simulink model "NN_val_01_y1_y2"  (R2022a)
settings: Solver=VariableStepAuto  StartTime=0.0  StopTime=300  RelTol=1e-3
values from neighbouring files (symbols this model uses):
  C = 6.3000e-04    (= 0.00063)    [maglev_init.m]
  g = 9.80    (= 9.8)    [maglev_init.m]
  K = 1.0e+03 * [-2.4567   -0.1235    0.0237]    [maglev_init.m]
  L1 = 0.6000    (= 0.6)    [maglev_init.m]
  m = 0.0300    (= 0.03)    [maglev_init.m]
  mpert = 0    [maglev_init.m]
  R = 45    [maglev_init.m]
  Ts = 0.005    [maglev_init.m]    (also in train_net.m)
  x1_0 = 0.1    [maglev_init.m]
  x1_d = 0.05    [maglev_init.m]
  x2_0 = 0    [maglev_init.m]
  x2_d = 0    [maglev_init.m]
  x3_0 = 0.2    [maglev_init.m]
undefined symbols (not defined in the file or in its folder): magnitude
libraries: neural x26

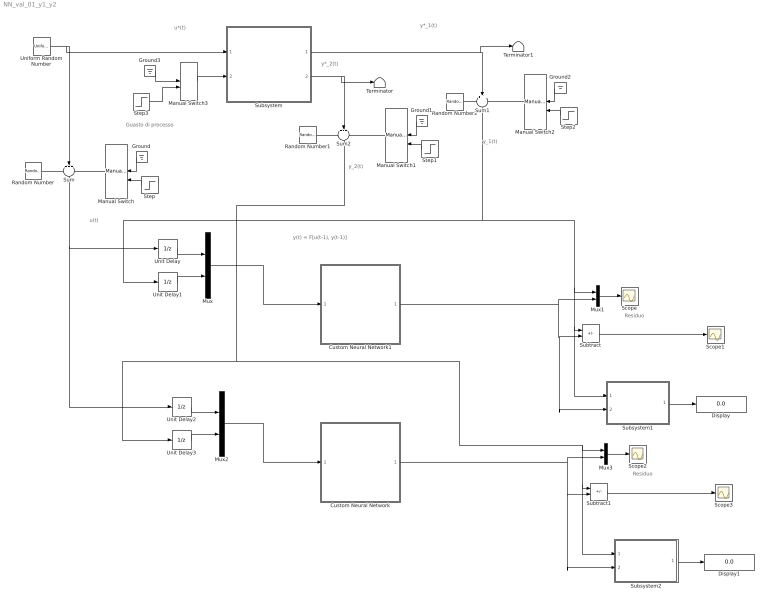
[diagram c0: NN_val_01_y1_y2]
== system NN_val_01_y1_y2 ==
  note: Residuo
  note: y(t) = F[u(t-1), y(t-1)]
  note: y_2(t)
  note: y*_1(t)
  note: u(t)
  note: y*_2(t)
  note: y_1(t)
  note: u*(t)
  note: Guasto di processo
  note: Residuo
  Custom Neural Network : Subsystem
      mask help: Custom Neural Network
  Custom Neural Network1 : Subsystem
      mask help: Custom Neural Network
  Display : Display
  Display1 : Display
  Ground{,1..3} (4 alike) : Ground
  Manual Switch : ManualSwitch
  Manual Switch1 : ManualSwitch  CurrentSetting=0
  Manual Switch2 : ManualSwitch
  Manual Switch3 : ManualSwitch
  Mux{,1..3} (4 alike) : Mux  Inputs=2
  Random Number : RandomNumber  Variance=1e-9  Seed=1  SampleTime=Ts
  Random Number1 : RandomNumber  Variance=1e-6  Seed=3  SampleTime=Ts
  Random Number2 : RandomNumber  Variance=1e-9  Seed=2  SampleTime=Ts
  Scope{,1..3} (4 alike) : Scope
  Step : Step  Time=150  SampleTime=0
  Step1 : Step  Time=150  SampleTime=0
  Step2 : Step  Time=150  SampleTime=0
  Step3 : Step  Time=15  After=2*R  SampleTime=0
  Subsystem : Subsystem
  Subsystem1 : Subsystem
  Subsystem2 : Subsystem
  Subtract : Sum  Inputs=+-
  Subtract1 : Sum  Inputs=+-
  Sum : Sum  Inputs=+++
  Sum1 : Sum  Inputs=+++
  Sum2 : Sum  Inputs=+++
  Terminator : Terminator
  Terminator1 : Terminator
  Uniform Random Number : UniformRandomNumber  Minimum=x1_d*0.9  Maximum=x1_d*1.1  Seed=1  SampleTime=0.5
  Unit Delay{,1..3} (4 alike) : UnitDelay  SampleTime=Ts  HasFrameUpgradeWarning=on
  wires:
  Subsystem/1(Out1) -> Terminator1/1, Sum1/2
  Subsystem/2(Out2) -> Terminator/1, Sum2/2
  Random Number/1 -> Sum/1
  Manual Switch/1 -> Sum/3
  Manual Switch2/1 -> Sum1/3
  Manual Switch1/1 -> Sum2/3
  Random Number1/1 -> Sum2/1
  Ground/1 -> Manual Switch/1
  Step/1 -> Manual Switch/2
  Ground1/1 -> Manual Switch1/1
  Step1/1 -> Manual Switch1/2
  Random Number2/1 -> Sum1/1
  Ground2/1 -> Manual Switch2/1
  Step2/1 -> Manual Switch2/2
  Manual Switch3/1 -> Subsystem/2(fs)
  Ground3/1 -> Manual Switch3/1
  Uniform Random Number/1 -> Subsystem/1(u), Sum/2
  Step3/1 -> Manual Switch3/2
  Sum/1 -> Unit Delay2/1, Unit Delay/1
  Unit Delay/1 -> Mux/1
  Unit Delay1/1 -> Mux/2
  Mux/1 -> Custom Neural Network1/1(Input)
  Custom Neural Network1/1(Output) -> Mux1/2, Subsystem1/2(y_prev), Subtract/2
  Subtract/1 -> Scope1/1
  Mux1/1 -> Scope/1
  Sum1/1 -> Subsystem1/1(y_mis), Subtract/1, Mux1/1, Unit Delay1/1
  Subsystem1/1(VAF%) -> Display/1
  Mux2/1 -> Custom Neural Network/1(Input)
  Unit Delay2/1 -> Mux2/1
  Unit Delay3/1 -> Mux2/2
  Subtract1/1 -> Scope3/1
  Custom Neural Network/1(Output) -> Mux3/2, Subsystem2/2(y_prev), Subtract1/2
  Mux3/1 -> Scope2/1
  Subsystem2/1(VAF%) -> Display1/1
  Sum2/1 -> Subsystem2/1(y_mis), Subtract1/1, Mux3/1, Unit Delay3/1

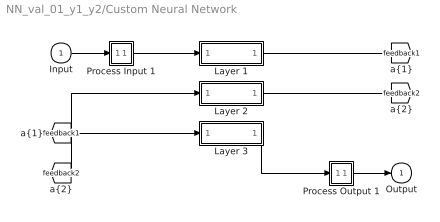
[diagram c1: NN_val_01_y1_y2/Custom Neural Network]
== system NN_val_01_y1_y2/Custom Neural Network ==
  Input : Inport  PortDimensions=2  SampleTime=0.005
  Layer 1 : Subsystem
  Layer 2 : Subsystem
  Layer 3 : Subsystem
  Process Input 1 : Subsystem
  Process Output 1 : Subsystem
  Output : Outport  InitialOutput=0
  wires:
  Input/1 -> Process Input 1/1(x)
  Process Output 1/1(y) -> Output/1
  Process Input 1/1(p) -> Layer 1/1("p{1}")
  Layer 1/1("a{1}") -> [feedback1]
  [feedback1] -> Layer 2/1("a{1} ")
  Layer 2/1("a{2}") -> [feedback2]
  [feedback2] -> Layer 3/1("a{2} ")
  Layer 3/1("a{3}") -> Process Output 1/1(a)

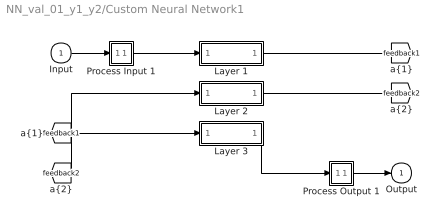
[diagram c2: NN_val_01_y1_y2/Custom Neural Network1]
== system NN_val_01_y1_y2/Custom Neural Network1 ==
  Input : Inport  PortDimensions=2  SampleTime=0.005
  Layer 1 : Subsystem
  Layer 2 : Subsystem
  Layer 3 : Subsystem
  Process Input 1 : Subsystem
  Process Output 1 : Subsystem
  Output : Outport  InitialOutput=0
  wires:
  Layer 3/1("a{3}") -> Process Output 1/1(a)
  [feedback2] -> Layer 3/1("a{2} ")
  Layer 2/1("a{2}") -> [feedback2]
  [feedback1] -> Layer 2/1("a{1} ")
  Layer 1/1("a{1}") -> [feedback1]
  Process Input 1/1(p) -> Layer 1/1("p{1}")
  Process Output 1/1(y) -> Output/1
  Input/1 -> Process Input 1/1(x)

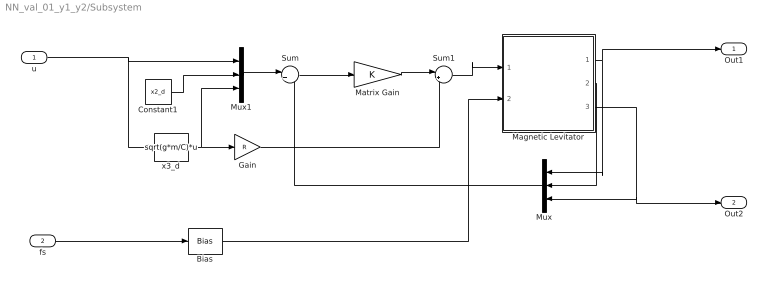
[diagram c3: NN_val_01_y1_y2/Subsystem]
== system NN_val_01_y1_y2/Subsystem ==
  u : Inport
  fs : Inport  Port=2
  Bias : Bias  Bias=R
  Constant1 : Constant  Value=x2_d
  Gain : Gain  Gain=R
  Magnetic Levitator : Subsystem  mask{m=m+mpert, R=R, L1=L1, C=C, g=g}
      mask prompts: m "ball's mass (m)"; R "Electromagnet's resistance (R)"; L1 "Electromagnet's inductance (L1)"; C "Magnetic force constant (C)"; g "Gravitational acceleration (g)"
  Matrix Gain : Gain  Gain=K  Multiplication=Matrix(K*u)  SaturateOnIntegerOverflow=on
  Mux : Mux  Inputs=3
  Mux1 : Mux  Inputs=3
  Sum : Sum  Inputs=|+-  InputSameDT=on  SaturateOnIntegerOverflow=on
  Sum1 : Sum  Inputs=|++  InputSameDT=on  SaturateOnIntegerOverflow=on
  x3_d : Fcn  Expr=sqrt(g*m/C)*u
  Out1 : Outport
  Out2 : Outport  Port=2
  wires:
  u/1 -> x3_d/1, Mux1/1
  Magnetic Levitator/2(x2) -> Mux/2
  x3_d/1 -> Mux1/3, Gain/1
  Mux1/1 -> Sum/1
  Gain/1 -> Sum1/2
  Mux/1 -> Sum/2
  Constant1/1 -> Mux1/2
  Sum/1 -> Matrix Gain/1
  Sum1/1 -> Magnetic Levitator/1(u)
  Magnetic Levitator/1(x1) -> Out1/1, Mux/1
  Magnetic Levitator/3(x3) -> Out2/1, Mux/3
  Matrix Gain/1 -> Sum1/1
  Bias/1 -> Magnetic Levitator/2(fs)
  fs/1 -> Bias/1

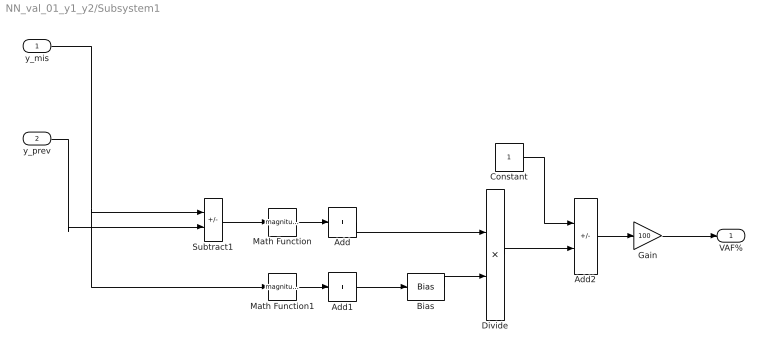
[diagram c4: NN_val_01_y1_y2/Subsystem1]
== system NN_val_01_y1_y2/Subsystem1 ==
  y_mis : Inport
  y_prev : Inport  Port=2
  Add : Sum  Inputs=+
  Add1 : Sum  Inputs=+
  Add2 : Sum  Inputs=+-
  Bias : Bias  Bias=1e-7
  Constant : Constant
  Divide : Product  Inputs=*/
  Gain : Gain  Gain=100
  Math Function : Math  Operator=magnitude^2
  Math Function1 : Math  Operator=magnitude^2
  Subtract1 : Sum  Inputs=+-
  VAF% : Outport
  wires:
  Add2/1 -> Gain/1
  Math Function/1 -> Add/1
  Bias/1 -> Divide/2
  y_mis/1 -> Math Function1/1, Subtract1/1
  Add1/1 -> Bias/1
  Math Function1/1 -> Add1/1
  Subtract1/1 -> Math Function/1
  Constant/1 -> Add2/1
  Divide/1 -> Add2/2
  Add/1 -> Divide/1
  y_prev/1 -> Subtract1/2
  Gain/1 -> VAF%/1

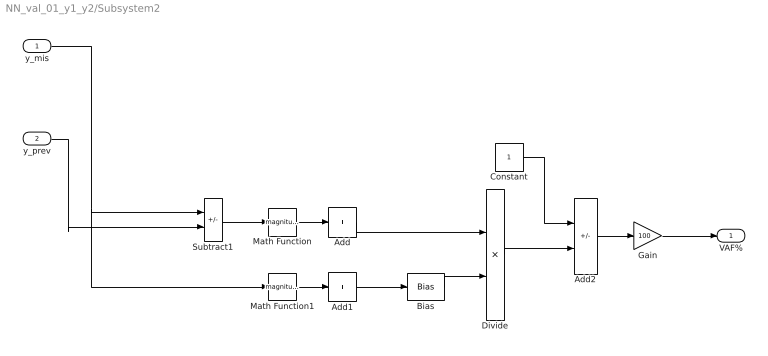
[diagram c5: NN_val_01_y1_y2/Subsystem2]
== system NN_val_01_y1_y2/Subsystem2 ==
  y_mis : Inport
  y_prev : Inport  Port=2
  Add : Sum  Inputs=+
  Add1 : Sum  Inputs=+
  Add2 : Sum  Inputs=+-
  Bias : Bias  Bias=1e-7
  Constant : Constant
  Divide : Product  Inputs=*/
  Gain : Gain  Gain=100
  Math Function : Math  Operator=magnitude^2
  Math Function1 : Math  Operator=magnitude^2
  Subtract1 : Sum  Inputs=+-
  VAF% : Outport
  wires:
  Add2/1 -> Gain/1
  Math Function/1 -> Add/1
  Bias/1 -> Divide/2
  y_mis/1 -> Math Function1/1, Subtract1/1
  Add1/1 -> Bias/1
  Math Function1/1 -> Add1/1
  Subtract1/1 -> Math Function/1
  Constant/1 -> Add2/1
  Divide/1 -> Add2/2
  Add/1 -> Divide/1
  y_prev/1 -> Subtract1/2
  Gain/1 -> VAF%/1

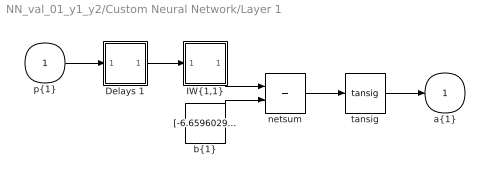
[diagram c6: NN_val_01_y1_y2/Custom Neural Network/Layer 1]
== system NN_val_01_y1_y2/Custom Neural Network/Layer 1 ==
  "p{1}" : Inport  PortDimensions=2  SampleTime=0.005
  Delays 1 : Subsystem
  "IW{1,1}" : Subsystem
  "b{1}" : Constant  Value=[-6.659602904330821360190384439192712306976318359375;3.45327763320656888623716440633870661258697509765625;1.7250442827917229493550621555186808109283447265625;0.2469389502636202549101795966635108925402164459228515625]
  netsum : Sum  Inputs=2  InputSameDT=on  SaturateOnIntegerOverflow=on
  tansig : neural/Transfer Functions/tansig
  "a{1}" : Outport  InitialOutput=[0;0;0;0]
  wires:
  "p{1}"/1 -> Delays 1/1("p{1}")
  Delays 1/1("pd{1,1}") -> "IW{1,1}"/1("pd{1,1}")
  "IW{1,1}"/1("iz{1,1}") -> netsum/1
  "b{1}"/1 -> netsum/2
  netsum/1 -> tansig/1
  tansig/1 -> "a{1}"/1

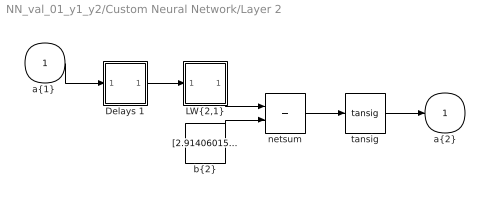
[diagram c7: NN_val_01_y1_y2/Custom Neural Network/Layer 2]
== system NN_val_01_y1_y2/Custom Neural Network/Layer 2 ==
  "a{1} " : Inport  PortDimensions=4  SampleTime=0.005
  Delays 1 : Subsystem
  "LW{2,1}" : Subsystem
  "b{2}" : Constant  Value=[2.914060157524335448187002839404158294200897216796875;-1.7057329147950757164409196775523014366626739501953125;-1.0860188396599046445345493339118547737598419189453125;-0.237937741106720890282844038665643893182277679443359375;-0.2127850090079609068904886726159020327031612396240234375;1.0101599307664710369891736263525672256946563720703125;1.8204085838934105368025484494864940643310546875;-2.778407191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
  netsum : Sum  Inputs=2  InputSameDT=on  SaturateOnIntegerOverflow=on
  tansig : neural/Transfer Functions/tansig
  "a{2}" : Outport  InitialOutput=[0;0;0;0;0;0;0;0]
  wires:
  "a{1} "/1 -> Delays 1/1("p{2}")
  Delays 1/1("pd{2,1}") -> "LW{2,1}"/1("ad{2,1}")
  "LW{2,1}"/1("lz{2,1}") -> netsum/1
  "b{2}"/1 -> netsum/2
  netsum/1 -> tansig/1
  tansig/1 -> "a{2}"/1

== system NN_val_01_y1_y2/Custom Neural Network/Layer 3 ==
  "a{2} " : Inport  PortDimensions=8  SampleTime=0.005
  Delays 1 : Subsystem
  "LW{3,2}" : Subsystem
  "b{3}" : Constant  Value=0.5176708554335636147669674755888991057872772216796875
  netsum : Sum  Inputs=2  InputSameDT=on  SaturateOnIntegerOverflow=on
  purelin : neural/Transfer Functions/purelin
  "a{3}" : Outport  InitialOutput=0
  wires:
  "a{2} "/1 -> Delays 1/1("p{3}")
  Delays 1/1("pd{3,2}") -> "LW{3,2}"/1("ad{3,2}")
  "LW{3,2}"/1("lz{3,2}") -> netsum/1
  "b{3}"/1 -> netsum/2
  netsum/1 -> purelin/1
  purelin/1 -> "a{3}"/1

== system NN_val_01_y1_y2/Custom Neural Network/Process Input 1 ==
  x : Inport  PortDimensions=2  SampleTime=0.005
  p : Outport  PortDimensions=2  SampleTime=0.005
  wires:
  x/1 -> p/1

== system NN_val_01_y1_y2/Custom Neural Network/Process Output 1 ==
  a : Inport  PortDimensions=1  SampleTime=0.005
  y : Outport  PortDimensions=1  SampleTime=0.005
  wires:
  a/1 -> y/1

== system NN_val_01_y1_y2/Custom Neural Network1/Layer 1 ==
  "p{1}" : Inport  PortDimensions=2  SampleTime=0.005
  Delays 1 : Subsystem
  "IW{1,1}" : Subsystem
  "b{1}" : Constant  Value=[-2.165010232984565075042837634100578725337982177734375;-0.99018084463472033629471980020753107964992523193359375]
  netsum : Sum  Inputs=2  InputSameDT=on  SaturateOnIntegerOverflow=on
  tansig : neural/Transfer Functions/tansig
  "a{1}" : Outport  InitialOutput=[0;0]
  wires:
  tansig/1 -> "a{1}"/1
  netsum/1 -> tansig/1
  "b{1}"/1 -> netsum/2
  "IW{1,1}"/1("iz{1,1}") -> netsum/1
  Delays 1/1("pd{1,1}") -> "IW{1,1}"/1("pd{1,1}")
  "p{1}"/1 -> Delays 1/1("p{1}")

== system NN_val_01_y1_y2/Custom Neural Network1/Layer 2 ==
  "a{1} " : Inport  PortDimensions=2  SampleTime=0.005
  Delays 1 : Subsystem
  "LW{2,1}" : Subsystem
  "b{2}" : Constant  Value=[-2.76409742947160541604034733609296381473541259765625;0.91391405324340713178798978333361446857452392578125;-0.79693396570784413857069239384145475924015045166015625;2.83340357653886432132139816530980169773101806640625]
  netsum : Sum  Inputs=2  InputSameDT=on  SaturateOnIntegerOverflow=on
  tansig : neural/Transfer Functions/tansig
  "a{2}" : Outport  InitialOutput=[0;0;0;0]
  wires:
  tansig/1 -> "a{2}"/1
  netsum/1 -> tansig/1
  "b{2}"/1 -> netsum/2
  "LW{2,1}"/1("lz{2,1}") -> netsum/1
  Delays 1/1("pd{2,1}") -> "LW{2,1}"/1("ad{2,1}")
  "a{1} "/1 -> Delays 1/1("p{2}")

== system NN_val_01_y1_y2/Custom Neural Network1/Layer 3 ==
  "a{2} " : Inport  PortDimensions=4  SampleTime=0.005
  Delays 1 : Subsystem
  "LW{3,2}" : Subsystem
  "b{3}" : Constant  Value=0.2010605623167778244209102922468446195125579833984375
  netsum : Sum  Inputs=2  InputSameDT=on  SaturateOnIntegerOverflow=on
  purelin : neural/Transfer Functions/purelin
  "a{3}" : Outport  InitialOutput=0
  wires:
  purelin/1 -> "a{3}"/1
  netsum/1 -> purelin/1
  "b{3}"/1 -> netsum/2
  "LW{3,2}"/1("lz{3,2}") -> netsum/1
  Delays 1/1("pd{3,2}") -> "LW{3,2}"/1("ad{3,2}")
  "a{2} "/1 -> Delays 1/1("p{3}")

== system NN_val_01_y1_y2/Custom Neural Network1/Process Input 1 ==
  x : Inport  PortDimensions=2  SampleTime=0.005
  p : Outport  PortDimensions=2  SampleTime=0.005
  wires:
  x/1 -> p/1

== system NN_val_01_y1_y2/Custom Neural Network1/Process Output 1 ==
  a : Inport  PortDimensions=1  SampleTime=0.005
  y : Outport  PortDimensions=1  SampleTime=0.005
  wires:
  a/1 -> y/1

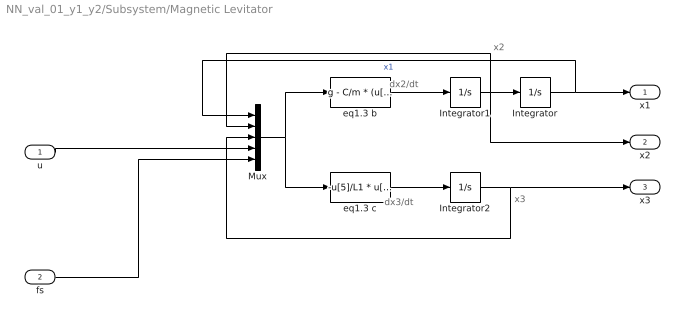
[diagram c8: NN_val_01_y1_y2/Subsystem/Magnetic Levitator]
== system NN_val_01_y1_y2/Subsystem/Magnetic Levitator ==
  note: x2
  note: x3
  note: dx2/dt
  note: dx3/dt
  u : Inport
  fs : Inport  Port=2
  Integrator : Integrator  InitialCondition=x1_0
  Integrator1 : Integrator  InitialCondition=x2_0
  Integrator2 : Integrator  InitialCondition=x3_0
  Mux : Mux  Inputs=5
  eq1.3 b : Fcn  Expr=g - C/m * (u[3] / u[1])^2
  eq1.3 c : Fcn  Expr=-u[5]/L1 * u[3] + (2*C)/L1 * ( u[2] * u[3] / u[1]^2 ) + 1/L1 * u[4]
  x1 : Outport
  x2 : Outport  Port=2
  x3 : Outport  Port=3
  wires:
  eq1.3 b/1 -> Integrator1/1
  Integrator1/1 -> Integrator/1, Mux/2, x2/1
  eq1.3 c/1 -> Integrator2/1
  Mux/1 -> eq1.3 b/1, eq1.3 c/1
  Integrator/1 -> Mux/1, x1/1  "x1"
  Integrator2/1 -> Mux/3, x3/1
  u/1 -> Mux/4
  fs/1 -> Mux/5

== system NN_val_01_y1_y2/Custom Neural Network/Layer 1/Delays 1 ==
  "p{1}" : Inport  PortDimensions=2  SampleTime=0.005
  mux : Mux  Inputs=1
  "pd{1,1}" : Outport
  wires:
  "p{1}"/1 -> mux/1
  mux/1 -> "pd{1,1}"/1

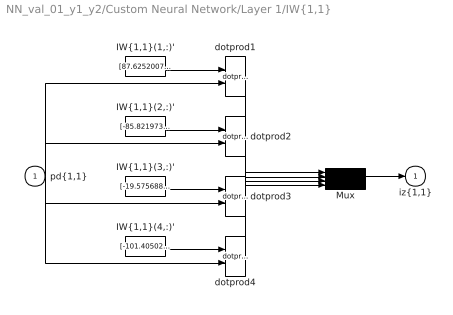
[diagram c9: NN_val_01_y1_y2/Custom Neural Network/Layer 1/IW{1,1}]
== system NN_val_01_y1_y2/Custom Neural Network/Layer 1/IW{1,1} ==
  "pd{1,1}" : Inport  PortDimensions=2  SampleTime=0.005
  "IW{1,1}(1,:)'" : Constant  Value=[87.6252007333225577667690231464803218841552734375;2.19082573935980828849778845324181020259857177734375]
  "IW{1,1}(2,:)'" : Constant  Value=[-85.8219734896255204148474149405956268310546875;0.669958335690548967278346026432700455188751220703125]
  "IW{1,1}(3,:)'" : Constant  Value=[-19.5756880526265462094670510850846767425537109375;-3.06946859135708383092833173577673733234405517578125]
  "IW{1,1}(4,:)'" : Constant  Value=[-101.405020836113436644154717214405536651611328125;-0.17119351877394961558565000814269296824932098388671875]
  Mux : Mux
  dotprod{1..4} (4 alike) : neural/Weight Functions/dotprod
  "iz{1,1}" : Outport
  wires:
  "IW{1,1}(1,:)'"/1 -> dotprod1/1
  "pd{1,1}"/1 -> dotprod1/2, dotprod2/2, dotprod3/2, dotprod4/2
  dotprod1/1 -> Mux/1
  "IW{1,1}(2,:)'"/1 -> dotprod2/1
  dotprod2/1 -> Mux/2
  "IW{1,1}(3,:)'"/1 -> dotprod3/1
  dotprod3/1 -> Mux/3
  "IW{1,1}(4,:)'"/1 -> dotprod4/1
  dotprod4/1 -> Mux/4
  Mux/1 -> "iz{1,1}"/1

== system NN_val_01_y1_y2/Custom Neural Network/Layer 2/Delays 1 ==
  "p{2}" : Inport  PortDimensions=4  SampleTime=0.005
  mux : Mux  Inputs=1
  "pd{2,1}" : Outport
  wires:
  "p{2}"/1 -> mux/1
  mux/1 -> "pd{2,1}"/1

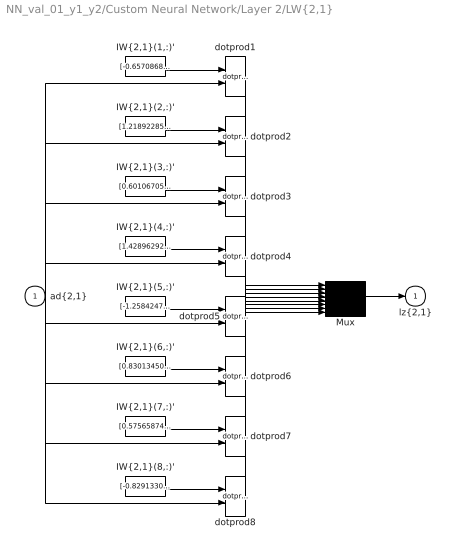
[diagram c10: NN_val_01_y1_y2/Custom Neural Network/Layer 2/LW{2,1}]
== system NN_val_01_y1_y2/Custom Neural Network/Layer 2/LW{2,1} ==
  "ad{2,1}" : Inport  PortDimensions=4  SampleTime=0.005
  "IW{2,1}(1,:)'" : Constant  Value=[-0.6570868886894183358293730634613893926143646240234375;-2.163165004665934976202379402820952236652374267578125;-0.5532020086247440016080645364127121865749359130859375;0.9859704403199989197759123271680437028408050537109375]
  "IW{2,1}(2,:)'" : Constant  Value=[1.2189228592566114794948362032300792634487152099609375;-0.7015962880393835643388911194051615893840789794921875;1.0463907528220131037954843122861348092555999755859375;-1.6363234229084560045208718292997218668460845947265625]
  "IW{2,1}(3,:)'" : Constant  Value=[0.60106705023984918767609997303225100040435791015625;1.4361829657222358047619081844459287822246551513671875;1.3759246081291902630283630060148425400257110595703125;1.1204977777650817483134915164555422961711883544921875]
  "IW{2,1}(4,:)'" : Constant  Value=[1.4289629233486953463483359882957302033901214599609375;-0.275198140282933767508666278445161879062652587890625;2.049677383815454501103658913052640855312347412109375;-1.096912197977354619382595046772621572017669677734375]
  "IW{2,1}(5,:)'" : Constant  Value=[-1.2584247288445358226027792625245638191699981689453125;0.531729868681150907860910592717118561267852783203125;0.020485692905892971538150959531776607036590576171875;1.92155818448143467236377546214498579502105712890625]
  "IW{2,1}(6,:)'" : Constant  Value=[0.830134509065694192742057566647417843341827392578125;-1.2880179778638976006988059452851302921772003173828125;-1.64143888892304534721233721938915550708770751953125;-0.69165869509857558217191808580537326633930206298828125]
  "IW{2,1}(7,:)'" : Constant  Value=[0.57565874445141940185521889361552894115447998046875;0.85671983433447496114609975847997702658176422119140625;-1.3194661778970104837327426139381714165210723876953125;-1.4686793163921338933874949361779727041721343994140625]
  "IW{2,1}(8,:)'" : Constant  Value=[-0.82913308009071418069879655377008020877838134765625;-0.78734936389389054145482305102632381021976470947265625;-0.95701288861991462564304811166948638856410980224609375;-0.65442341548820337493452825583517551422119140625]
  Mux : Mux  Inputs=8
  dotprod{1..8} (8 alike) : neural/Weight Functions/dotprod
  "lz{2,1}" : Outport
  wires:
  "IW{2,1}(1,:)'"/1 -> dotprod1/1
  "ad{2,1}"/1 -> dotprod1/2, dotprod2/2, dotprod3/2, dotprod4/2, dotprod5/2, dotprod6/2, dotprod7/2, dotprod8/2
  dotprod1/1 -> Mux/1
  "IW{2,1}(2,:)'"/1 -> dotprod2/1
  dotprod2/1 -> Mux/2
  "IW{2,1}(3,:)'"/1 -> dotprod3/1
  dotprod3/1 -> Mux/3
  "IW{2,1}(4,:)'"/1 -> dotprod4/1
  dotprod4/1 -> Mux/4
  "IW{2,1}(5,:)'"/1 -> dotprod5/1
  dotprod5/1 -> Mux/5
  "IW{2,1}(6,:)'"/1 -> dotprod6/1
  dotprod6/1 -> Mux/6
  "IW{2,1}(7,:)'"/1 -> dotprod7/1
  dotprod7/1 -> Mux/7
  "IW{2,1}(8,:)'"/1 -> dotprod8/1
  dotprod8/1 -> Mux/8
  Mux/1 -> "lz{2,1}"/1

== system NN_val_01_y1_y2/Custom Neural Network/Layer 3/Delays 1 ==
  "p{3}" : Inport  PortDimensions=8  SampleTime=0.005
  mux : Mux  Inputs=1
  "pd{3,2}" : Outport
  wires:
  "p{3}"/1 -> mux/1
  mux/1 -> "pd{3,2}"/1

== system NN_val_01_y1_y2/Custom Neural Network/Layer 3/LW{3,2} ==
  "ad{3,2}" : Inport  PortDimensions=8  SampleTime=0.005
  "IW{3,2}(1,:)'" : Constant  Value=[-1.358437454784370945759519599960185587406158447265625;-0.5979801633767445334655121769174002110958099365234375;-0.1898552103770739518662225009393296204507350921630859375;0.77745792876645813951341779102222062647342681884765625;-0.39943154859763974062758506988757289946079254150390625;0.1445055083431290021689363811674411408603191375732421875;0.71498418383863249214726920399698428809642791748046875;-0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
  Mux : Mux  Inputs=1
  dotprod1 : neural/Weight Functions/dotprod
  "lz{3,2}" : Outport
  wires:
  "IW{3,2}(1,:)'"/1 -> dotprod1/1
  "ad{3,2}"/1 -> dotprod1/2
  dotprod1/1 -> Mux/1
  Mux/1 -> "lz{3,2}"/1

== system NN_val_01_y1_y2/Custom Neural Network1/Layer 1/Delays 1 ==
  "p{1}" : Inport  PortDimensions=2  SampleTime=0.005
  mux : Mux  Inputs=1
  "pd{1,1}" : Outport
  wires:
  mux/1 -> "pd{1,1}"/1
  "p{1}"/1 -> mux/1

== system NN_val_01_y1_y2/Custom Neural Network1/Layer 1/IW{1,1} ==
  "pd{1,1}" : Inport  PortDimensions=2  SampleTime=0.005
  "IW{1,1}(1,:)'" : Constant  Value=[46.38752532641807846403025905601680278778076171875;-30.02020716206245509738437249325215816497802734375]
  "IW{1,1}(2,:)'" : Constant  Value=[50.408506029134514392353594303131103515625;28.00458439829532153453328646719455718994140625]
  Mux : Mux  Inputs=2
  dotprod1 : neural/Weight Functions/dotprod
  dotprod2 : neural/Weight Functions/dotprod
  "iz{1,1}" : Outport
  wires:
  Mux/1 -> "iz{1,1}"/1
  dotprod2/1 -> Mux/2
  "IW{1,1}(2,:)'"/1 -> dotprod2/1
  dotprod1/1 -> Mux/1
  "pd{1,1}"/1 -> dotprod2/2, dotprod1/2
  "IW{1,1}(1,:)'"/1 -> dotprod1/1

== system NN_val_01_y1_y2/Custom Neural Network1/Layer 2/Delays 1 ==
  "p{2}" : Inport  PortDimensions=2  SampleTime=0.005
  mux : Mux  Inputs=1
  "pd{2,1}" : Outport
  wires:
  mux/1 -> "pd{2,1}"/1
  "p{2}"/1 -> mux/1

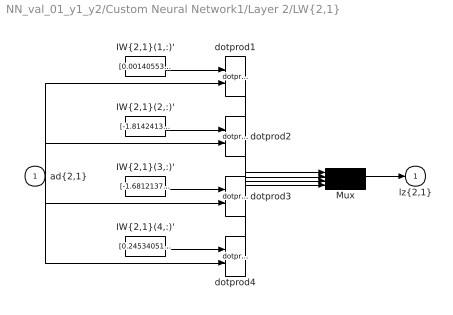
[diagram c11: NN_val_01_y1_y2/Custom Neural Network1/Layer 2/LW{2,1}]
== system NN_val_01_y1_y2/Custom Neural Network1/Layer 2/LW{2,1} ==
  "ad{2,1}" : Inport  PortDimensions=2  SampleTime=0.005
  "IW{2,1}(1,:)'" : Constant  Value=[0.001405533007920074795027431946436990983784198760986328125;2.76441434699151766807290186989121139049530029296875]
  "IW{2,1}(2,:)'" : Constant  Value=[-1.8142413042354241792253333187545649707317352294921875;2.12830136073460085555097975884564220905303955078125]
  "IW{2,1}(3,:)'" : Constant  Value=[-1.6812137832937150694334604850155301392078399658203125;-2.2096304124726291462366134510375559329986572265625]
  "IW{2,1}(4,:)'" : Constant  Value=[0.245340519136751533668672209387295879423618316650390625;2.76382363851122736519982936442829668521881103515625]
  Mux : Mux
  dotprod{1..4} (4 alike) : neural/Weight Functions/dotprod
  "lz{2,1}" : Outport
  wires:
  Mux/1 -> "lz{2,1}"/1
  dotprod4/1 -> Mux/4
  "IW{2,1}(4,:)'"/1 -> dotprod4/1
  dotprod3/1 -> Mux/3
  "IW{2,1}(3,:)'"/1 -> dotprod3/1
  dotprod2/1 -> Mux/2
  "IW{2,1}(2,:)'"/1 -> dotprod2/1
  dotprod1/1 -> Mux/1
  "ad{2,1}"/1 -> dotprod4/2, dotprod3/2, dotprod2/2, dotprod1/2
  "IW{2,1}(1,:)'"/1 -> dotprod1/1

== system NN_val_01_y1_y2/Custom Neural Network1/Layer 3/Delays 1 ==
  "p{3}" : Inport  PortDimensions=4  SampleTime=0.005
  mux : Mux  Inputs=1
  "pd{3,2}" : Outport
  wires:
  mux/1 -> "pd{3,2}"/1
  "p{3}"/1 -> mux/1

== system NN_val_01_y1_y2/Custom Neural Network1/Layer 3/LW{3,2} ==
  "ad{3,2}" : Inport  PortDimensions=4  SampleTime=0.005
  "IW{3,2}(1,:)'" : Constant  Value=[0.483295609205659226770279701668187044560909271240234375;0.356104986175123150449195463806972838938236236572265625;0.2319393811096205626487432027715840376913547515869140625;-0.2873034152097859728058892869739793241024017333984375]
  Mux : Mux  Inputs=1
  dotprod1 : neural/Weight Functions/dotprod
  "lz{3,2}" : Outport
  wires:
  Mux/1 -> "lz{3,2}"/1
  dotprod1/1 -> Mux/1
  "ad{3,2}"/1 -> dotprod1/2
  "IW{3,2}(1,:)'"/1 -> dotprod1/1
